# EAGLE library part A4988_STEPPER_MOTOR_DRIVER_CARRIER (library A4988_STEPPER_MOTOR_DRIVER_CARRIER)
Stepper motor controler; IC: A4988; 1A; Uin mot: 8÷35V
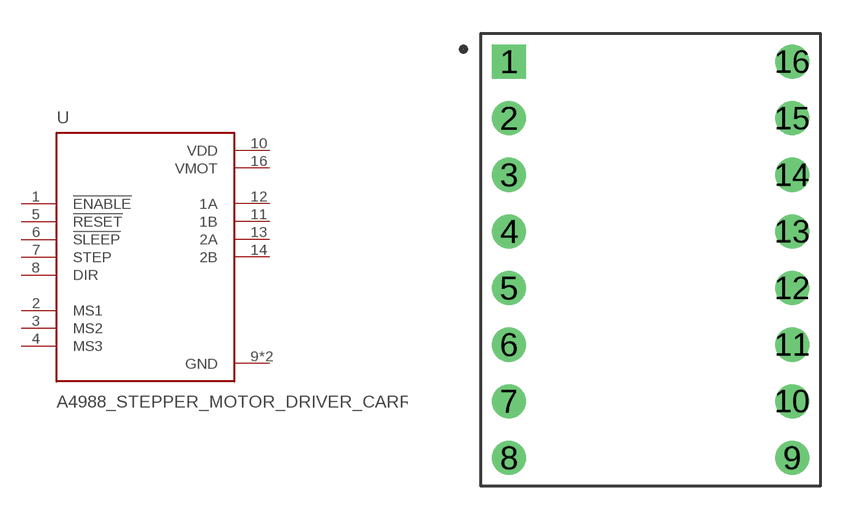
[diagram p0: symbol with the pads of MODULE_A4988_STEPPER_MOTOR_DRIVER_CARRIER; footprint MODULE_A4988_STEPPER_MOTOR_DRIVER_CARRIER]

Designator prefix U

## A4988_STEPPER_MOTOR_DRIVER_CARRIER (Availability: Unavailable; Description: Stepper Motor Driver; MF: Pololu; MP: A4988 STEPPER MOTOR DRIVER CARRIER; Package: None; Price: None)  [MODULE_A4988_STEPPER_MOTOR_DRIVER_CARRIER]
1  !ENABLE  in
2  MS1  in
3  MS2  in
4  MS3  in
5  !RESET  in
6  !SLEEP  in
7  STEP  in
8  DIR  in
9  GND  pwr
10  VDD  pwr
11  1B  out
12  1A  out
13  2A  out
14  2B  out
15  GND  pwr
16  VMOT  pwr

## Footprint MODULE_A4988_STEPPER_MOTOR_DRIVER_CARRIER (pad centres in mm)
drill 1.02 square: 1 -6.35,8.89
drill 1.02: 2 -6.35,6.35; 3 -6.35,3.81; 4 -6.35,1.27; 5 -6.35,-1.27; 6 -6.35,-3.81; 7 -6.35,-6.35; 8 -6.35,-8.89; 9 6.35,-8.89; 10 6.35,-6.35; 11 6.35,-3.81; 12 6.35,-1.27; 13 6.35,1.27; 14 6.35,3.81; 15 6.35,6.35; 16 6.35,8.89

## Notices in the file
This work is licensed under a Creative Commons Attribution-ShareAlike 4.0 International License (CC BY-SA) with Design Exception 1.0
